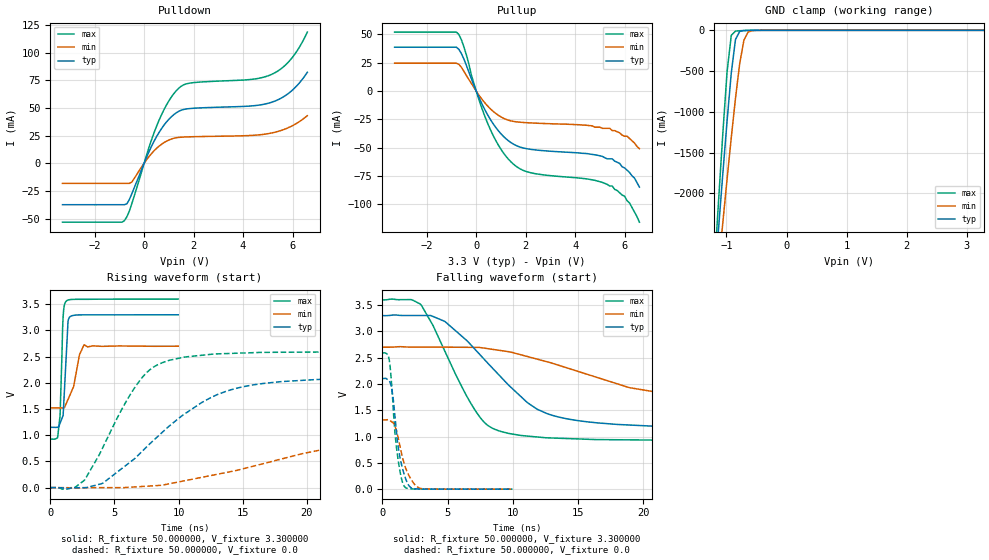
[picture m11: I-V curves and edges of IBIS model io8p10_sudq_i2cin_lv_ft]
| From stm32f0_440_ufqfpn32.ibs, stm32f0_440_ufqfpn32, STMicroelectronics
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|   Model io8p10_sudq_i2cin_lv_ft
[Model]  io8p10_sudq_i2cin_lv_ft
Model_type I/O
Polarity   Non-Inverting
Enable   Active-Low
Vinl =   0.990000V
Vinh =   2.310000V
Vmeas =  1.650000V
Cref =   50.000000pF
Rref =   100.000000M
Vref =   0.0V
C_comp   2.070000pF   1.996000pF   2.160200pF
[Temperature Range]   25.000000   0.125000k   -40.000000
[Pullup Reference]   3.300000V   2.700000V   3.600000V
[Pulldown Reference]   0.0V   0.0V   0.0V
[POWER Clamp Reference]   3.300000V   2.700000V   3.600000V
[GND Clamp Reference]   0.0V   0.0V   0.0V
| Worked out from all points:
|   slope of the pulldown table from 0 to 0.495 V, typ, clamps not added: 20.9 ohm
|   slope of the pullup table from 0 to 0.495 V, typ, clamps not added: 22.2 ohm
|   GND clamp passes 1 mA (typ) near -0.64 V on its own axis
|   rising waveform, R_fixture 50.000000, V_fixture 3.300000: 20-80 % time 274ps typ, 706ps min, 192ps max; typ from 1.15 V to 3.3 V
|   rising waveform, R_fixture 50.000000, V_fixture 0.0: 20-80 % time 6.37ns typ, 15ns min, 3.5ns max; typ from 0 V to 2.1 V
|   falling waveform, R_fixture 50.000000, V_fixture 3.300000: 20-80 % time 5.24ns typ, 11.1ns min, 3.25ns max; typ from 3.3 V to 1.15 V
|   falling waveform, R_fixture 50.000000, V_fixture 0.0: 20-80 % time 671ps typ, 884ps min, 550ps max; typ from 2.1 V to 0 V
[Pulldown]
|Voltage   I(typ)   I(min)   I(max)
-3.3V     -37.45mA   -18.2mA    -53.24mA
-800mV    -37.45mA   -18.2mA    -51.9mA
-700mV    -36.7mA    -18.2mA    -48.48mA
-500mV    -27.71mA   -17.01mA   -36.66mA
200mV     10.57mA    6.084mA    14.57mA
500mV     23.91mA    13.38mA    33.24mA
900mV     37.17mA    19.87mA    52.48mA
1.3V      45.55mA    23.01mA    65.5mA
1.8V      49.29mA    23.83mA    72.18mA
5.1V      54.68mA    27.07mA    79.72mA
5.9V      64.2mA     32.82mA    93.01mA
6.6V      82.13mA    42.97mA    118.4mA
[Pullup]
|Voltage   I(typ)   I(min)   I(max)
-3.3V     38.73mA    24.6mA     52.09mA
-800mV    38.73mA    24.6mA     52.09mA
-500mV    28.38mA    17.49mA    39.19mA
0V        90fA       16.1pA     0A
500mV     -22.5mA    -14.16mA   -30.52mA
900mV     -35.28mA   -21.55mA   -48mA
1.4V      -45.54mA   -26.4mA    -62.53mA
2.2V      -51.57mA   -28.22mA   -72.25mA
4.6V      -55.8mA    -30.6mA    -78.19mA
5.5V      -60mA      -35mA      -84mA
6V        -68mA      -40mA      -93mA
6.6V      -85mA      -51mA      -116mA
[GND_clamp]
|Voltage   I(typ)   I(min)   I(max)
-3.3V     -9.366A    -9.678A    -9.859A
-1.2V     -3.091A    -3.431A    -2.911A
-1.13V    -2.415A    -2.888A    -2.072A
-1.06V    -1.751A    -2.352A    -1.259A
-990mV    -1.112A    -1.826A    -509.3mA
-920mV    -522.9mA   -1.315A    -61.61mA
-850mV    -112.5mA   -833.8mA   -10.22mA
-780mV    -13.59mA   -408.1mA   -5.256mA
-710mV    -3.081mA   -122.1mA   -2.635mA
-640mV    -945.2uA   -21.36mA   -905.7uA
-570mV    -199.6uA   -4.142mA   -156.8uA
3.28V     0A         0A         0A
[POWER_clamp]
|Voltage   I(typ)   I(min)   I(max)
-3.28V    0A         0A         0A
0V        0A         0A         0A
[Ramp]
| variable   typ   min   max
dV/dt_r  1.26216/6.35979n   0.77952/15.03917n   1.55472/3.49910n
dV/dt_f  1.28946/5.23392n   0.69870/11.16902n   1.60471/3.24541n
R_load = 50.000000
[Rising Waveform]
R_fixture= 50.000000
V_fixture= 3.300000
V_fixture_min= 2.700000
V_fixture_max= 3.600000
|time   V(typ)   V(min)   V(max)
0s        1.151V     1.522V     925.5mV
580.6ps   1.153V     1.522V     976.8mV
760.8ps   1.228V     1.521V     1.37V
1.001ns   1.379V     1.522V     3.263V
1.221ns   2.412V     1.593V     3.556V
1.401ns   3.201V     1.694V     3.582V
1.822ns   3.289V     1.933V     3.594V
2.282ns   3.297V     2.543V     3.595V
2.643ns   3.298V     2.726V     3.595V
9.97ns    3.3V       2.7V       3.6V
[Rising Waveform]
R_fixture= 50.000000
V_fixture= 0.0
V_fixture_min= 0.0
V_fixture_max= 0.0
|time   V(typ)   V(min)   V(max)
0s        -32.6uV    -22.87uV   -20.68uV
2.603ns   -276.1uV   -5.444mV   128.9mV
4.104ns   86.95mV    -432.6uV   771.8mV
7.107ns   681.1mV    20.9mV     2.087V
8.308ns   961.6mV    39.17mV    2.339V
10.41ns   1.397V     128.5mV    2.491V
13.71ns   1.841V     289.1mV    2.559V
18.12ns   2.026V     553.4mV    2.584V
30.23ns   2.098V     1.113V     2.592V
49.85ns   2.104V     1.316V     2.591V
[Falling Waveform]
R_fixture= 50.000000
V_fixture= 3.300000
V_fixture_min= 2.700000
V_fixture_max= 3.600000
|time   V(typ)   V(min)   V(max)
0s        3.3V       2.7V       3.6V
2.903ns   3.303V     2.701V     3.522V
4.805ns   3.188V     2.701V     2.618V
7.307ns   2.606V     2.697V     1.43V
8.208ns   2.365V     2.668V     1.192V
9.71ns    1.973V     2.613V     1.059V
12.61ns   1.439V     2.424V     976.8mV
16.52ns   1.26V      2.122V     942.9mV
24.32ns   1.179V     1.71V      927.1mV
49.85ns   1.151V     1.522V     925.5mV
[Falling Waveform]
R_fixture= 50.000000
V_fixture= 0.0
V_fixture_min= 0.0
V_fixture_max= 0.0
|time   V(typ)   V(min)   V(max)
0s        2.104V     1.316V     2.591V
520.5ps   2.063V     1.315V     2.47V
760.8ps   1.847V     1.273V     1.818V
940.9ps   1.446V     1.208V     1.148V
1.081ns   1.094V     1.118V     797.7mV
1.421ns   521.5mV    735.2mV    252.7mV
1.722ns   245.1mV    451.2mV    40.86mV
2.142ns   38.17mV    211.3mV    6.468mV
2.883ns   3.131mV    17.1mV     2.592mV
9.97ns    -32.6uV    -22.87uV   -20.68uV
